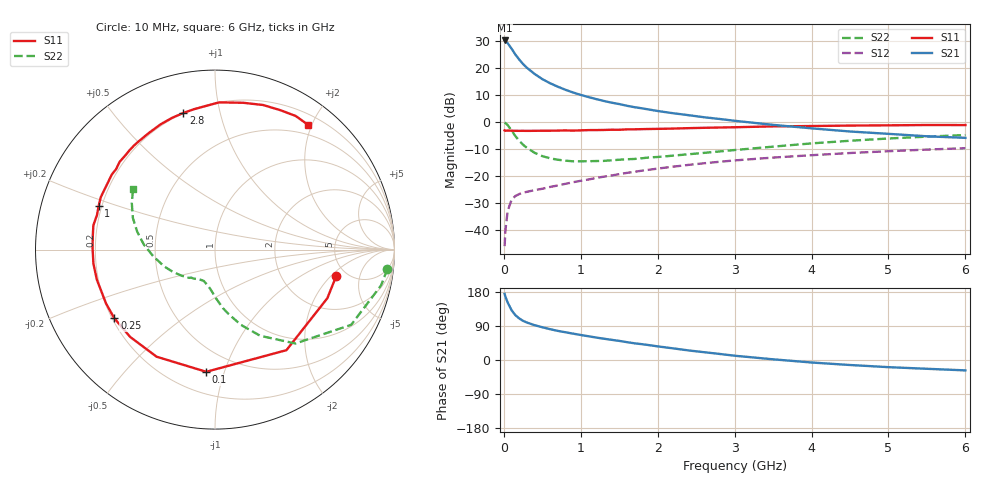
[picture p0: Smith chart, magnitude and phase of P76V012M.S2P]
! SIEMENS Small Signal Semiconductors
! BFP196
! Si NPN RF Bipolar Junction Transistor in SOT143
! VCE = 6 V  IC = 12 mA
! Common Emitter S-Parameters:  May  1996
# GHz  S  MA  R  50
!  f  S11  S21  S12  S22
! GHz  MAG  ANG  MAG  ANG  MAG  ANG  MAG  ANG
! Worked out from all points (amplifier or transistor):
!   36 points, 10 MHz to 6 GHz, reference 50 ohm
!   highest |S21| = 30.1 dB at 10 MHz (marker M1)
!   |S21| within 3 dB of that: start of sweep to 99.41 MHz
!   unconditionally stable (mu >= 1): 848.1 MHz to 3.302 GHz
!   at 250 MHz: K = 0.44, MSG = 23.8 dB, |S12| = -26.2 dB
!   at 1.4 GHz: K = 1.13, MAG = 11.3 dB, |S12| = -19.9 dB
!   at 6 GHz: K = 0.96, MSG = 1.9 dB, |S12| = -9.8 dB
!   S11 on the Smith chart (normalised r, x): 10 MHz: 4.13, -2.31; 100 MHz: 0.34, -0.87; 250 MHz: 0.21, -0.30; 1 GHz: 0.19, +0.18; 2.8 GHz: 0.20, +0.78; 6 GHz: 0.35, +1.94
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0.01  0.6916 -12.2  31.84 174.5  0.005 86.8  0.967 -6.4
0.02  0.682 -23.4  30.94 167.5  0.0097 81.1  0.9463 -12.2
0.05  0.6873 -54.6  28.36 151.6  0.0225 65.7  0.8669 -28.9
0.1  0.6825 -94.1  22.48 131.5  0.0358 50.6  0.6889 -49.4
0.15  0.6797 -118.6  17.5 118.2  0.0424 41.9  0.5425 -62.3
0.2  0.6784 -134.2  14.14 109.7  0.046 37.8  0.4444 -70.9
0.25  0.679 -145.7  11.66 103.3  0.0488 35.9  0.3745 -77.3
0.3  0.6772 -153.7  9.946 98.8  0.0506 35.3  0.3292 -82.3
0.4  0.6794 -165.8  7.644 91.9  0.0543 35.7  0.2665 -89.5
0.5  0.6819 -173.5  6.141 86.4  0.0576 37.1  0.2312 -94.7
0.6  0.6823 179.2  5.161 81.4  0.0622 39.0  0.211 -99.3
0.7  0.6854 173.3  4.456 76.9  0.0662 40.3  0.1985 -103.4
0.8  0.6911 168.7  3.903 73.2  0.0711 41.8  0.1907 -107.0
1  0.6925 159.3  3.132 66.0  0.0809 43.7  0.1853 -112.2
1.1  0.7002 155.4  2.861 62.6  0.0855 44.7  0.1862 -115.0
1.6  0.7221 137.4  1.972 47.1  0.1133 45.6  0.2023 -128.0
2.2  0.7475 119.3  1.436 30.7  0.1476 42.7  0.2361 -141.9
2.8  0.7816 103.0  1.127 16.1  0.1815 37.4  0.2819 -157.4
3.5  0.8206 88.4  0.875 1.8  0.2173 29.8  0.3462 -173.9
4.5  0.849 71.6  0.66 -13.2  0.264 19.1  0.445 167.0
5.5  0.8697 58.9  0.538 -23.2  0.3055 8.0  0.5304 150.9
6  0.8674 53.3  0.503 -27.4  0.3244 2.0  0.5677 143.6
